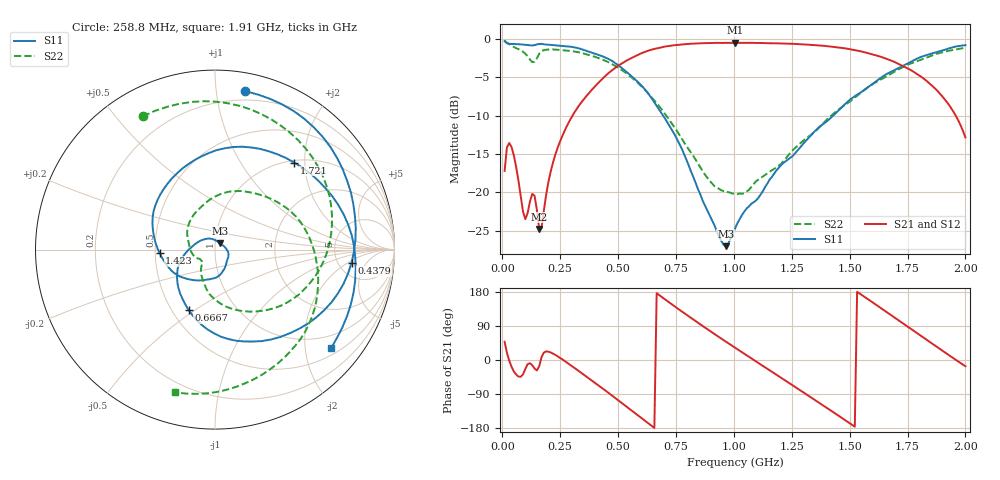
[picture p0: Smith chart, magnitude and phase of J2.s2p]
!Agilent Technologies,E8364B,MY43040703,A.07.50.48
!Agilent E8364B: A.07.50.48
!Date: Friday, November 12, 2021 03:03:23
!Correction: S11(Full 2 Port(1,2))
!S21(Full 2 Port(1,2))
!S12(Full 2 Port(1,2))
!S22(Full 2 Port(1,2))
!S2P File: Measurements: S11, S21, S12, S22:
# Hz S  RI  R 50
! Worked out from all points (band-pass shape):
!   201 points, 10 MHz to 2 GHz, reference 50 ohm
!   highest |S21| = -0.51 dB at 1.005 GHz (marker M1); lowest = -24.8 dB at 159.2 MHz (marker M2)
!   |S21| within 3 dB of the highest: 500.8 MHz to 1.728 GHz (1.227 GHz wide, 110 % of centre)
!   lowest |S11| = -27.0 dB at 965.2 MHz (marker M3), VSWR 1.09, Z = 52.7 + j3.67 ohm
!   |S11| at or under -10 dB: 694.6 MHz to 1.429 GHz (734.5 MHz wide, 69.2 % of centre)
!   |S22| runs from -20.2 to -0.2 dB; largest |S21 - S12| = 0.0022
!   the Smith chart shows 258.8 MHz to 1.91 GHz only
!   S11 on the Smith chart (normalised r, x): 258.8 MHz: 0.13, +1.20; 437.9 MHz: 6.64, -2.35; 666.7 MHz: 0.61, -0.47; 1.423 GHz: 0.53, -0.02; 1.721 GHz: 1.04, +1.77; 1.91 GHz: 0.65, -2.57
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1e7  0.5299 -0.8094  0.092 0.1026  0.0922 0.1032  0.8956 -0.3901
2.99e7  -0.5 -0.783  0.2095 -0.00659  0.2096 -0.00727  0.4132 -0.8268
4.98e7  -0.8377 -0.3961  0.1507 -0.0874  0.1507 -0.0875  -0.0948 -0.8813
8.96e7  -0.9017 0.1766  0.0589 -0.0457  0.0589 -0.0457  -0.6677 -0.4835
1.5925e8  -0.5862 0.7182  0.0551 -0.0168  0.0549 -0.0167  -0.7976 0.0418
2.5875e8  0.1657 0.8833  0.2316 0.00778  0.2315 0.0076  -0.4016 0.7427
3.483e8  0.6797 0.5116  0.3167 -0.2403  0.3168 -0.2402  0.2007 0.7802
4.3785e8  0.7607 -0.0736  0.1255 -0.5454  0.1251 -0.5456  0.5999 0.4116
5.473e8  0.3115 -0.5012  -0.4563 -0.578  -0.4557 -0.5781  0.5594 -0.1473
6.667e8  -0.1472 -0.3357  -0.8654 0.0559  -0.8653 0.0561  0.1644 -0.3433
6.7665e8  -0.1654 -0.3057  -0.8648 0.1252  -0.8645 0.1253  0.1349 -0.3397
8.259e8  -0.123 0.0209  -0.2609 0.8934  -0.2616 0.8948  -0.0726 -0.1555
9.652e8  0.0279 0.0347  0.6224 0.7078  0.6211 0.7064  -0.0696 -0.0745
1.005e9  0.0571 0.0108  0.7947 0.5085  0.7938 0.5083  -0.0747 -0.0627
1.15425e9  0.0511 -0.1094  0.8348 -0.4253  0.8339 -0.4258  -0.1362 -0.00407
1.3433e9  -0.1922 -0.1516  -0.2006 -0.8893  -0.2008 -0.8902  -0.0871 0.2276
1.4229e9  -0.3091 -0.0191  -0.6293 -0.6292  -0.6298 -0.6291  0.0469 0.3146
1.5423e9  -0.286 0.3373  -0.8311 0.0611  -0.8299 0.0613  0.3496 0.2634
1.67165e9  0.1984 0.5693  -0.3816 0.6221  -0.3813 0.6217  0.5728 -0.1187
1.7214e9  0.4419 0.4845  -0.1235 0.6632  -0.1228 0.6636  0.5548 -0.3288
1.91045e9  0.646 -0.5505  0.3788 0.1415  0.3789 0.1415  -0.2229 -0.7948
2e9  0.1174 -0.9028  0.2186 -0.0643  0.2186 -0.0643  -0.7139 -0.5074
